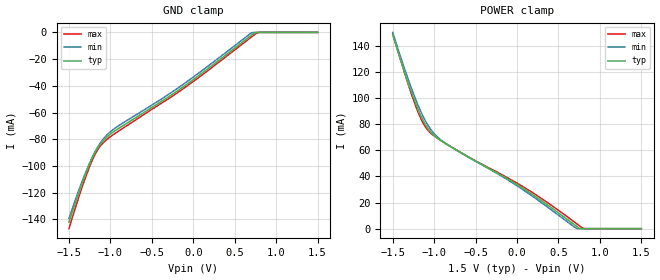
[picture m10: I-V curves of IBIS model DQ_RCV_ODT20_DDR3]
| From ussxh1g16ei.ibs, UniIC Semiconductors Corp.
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|   Model DQ_RCV_ODT20_DDR3
[Model] DQ_RCV_ODT20_DDR3
Model_type Input
Vinl =  0.615V
Vinh =  0.885V
C_comp   1.232pF   1.219pF   1.235pF
[Model Spec]
Vinh   0.885V   0.847V   0.922V
Vinl   0.615V   0.577V   0.652V
[Temperature Range]   25.000   95.000   -40.000
[Voltage Range]   1.500V   1.425V   1.575V
[GND_clamp]
|Voltage   I(typ)   I(min)   I(max)
-1.5V     -142mA     -139.3mA   -146.9mA
-1.345V   -113.6mA   -112.1mA   -116.5mA
-1.283V   -103.4mA   -102.4mA   -105.6mA
-1.221V   -94.43mA   -93.69mA   -95.96mA
-1.128V   -84.14mA   -83.3mA    -85.5mA
-1.035V   -77.85mA   -76.32mA   -79.73mA
-911mV    -72.33mA   -70.28mA   -74.3mA
-136mV    -41.39mA   -39.51mA   -42.79mA
701mV     -2.131mA   -333uA     -3.521mA
732mV     -645.7uA   0A         -2.04mA
794mV     0A         0A         0A
1.5V      0A         0A         0A
[POWER_clamp]
|Voltage   I(typ)   I(min)   I(max)
-1.5V     148.6mA    150.3mA    149.5mA
-1.321V   113mA      115.9mA    112.1mA
-1.197V   91.69mA    94.99mA    89.68mA
-1.104V   79.54mA    82.4mA     77.78mA
-1.011V   72.02mA    73.58mA    71.49mA
-918mV    67.43mA    67.95mA    67.47mA
-794mV    62.54mA    62.52mA    62.67mA
105mV     29.61mA    28.39mA    30.89mA
725mV     1.411mA    0A         3.569mA
756mV     0A         0A         2.101mA
818mV     0A         0A         0A
1.5V      0A         0A         0A
